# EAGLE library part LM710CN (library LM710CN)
Analog Comparators Source: Datasheet
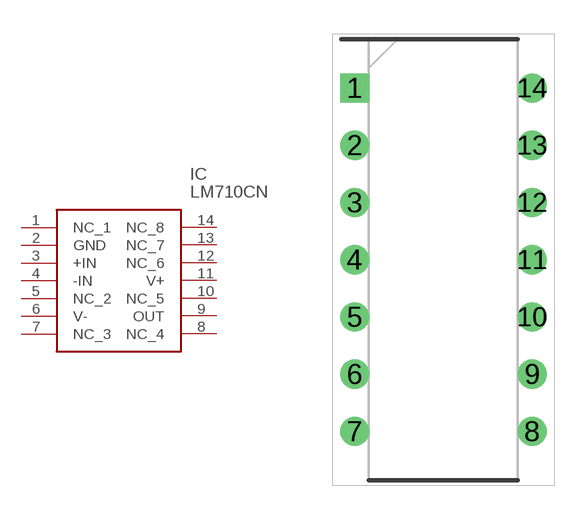
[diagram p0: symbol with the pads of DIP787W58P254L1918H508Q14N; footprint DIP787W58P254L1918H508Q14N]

Designator prefix IC

## LM710CN (Description: Analog Comparators; Height: 5.08mm; Manufacturer_Name: Texas Instruments; Manufacturer_Part_Number: LM710CN; Mouser_Part_Number: N/A; Mouser_Price-Stock: https://www.mouser.com/Search/Refine.aspx?Keyword=N%2FA)  [DIP787W58P254L1918H508Q14N]
1  NC_1
2  GND
3  +IN
4  -IN
5  NC_2
6  V-
7  NC_3
8  NC_4
9  OUT
10  NC_5
11  V+
12  NC_6
13  NC_7
14  NC_8

## Footprint DIP787W58P254L1918H508Q14N (pad centres in mm)
N14A
drill 0.784 pad 1.184 square: 1 -3.937,7.62
drill 0.784 pad 1.184: 2 -3.937,5.08; 3 -3.937,2.54; 4 -3.937,0; 5 -3.937,-2.54; 6 -3.937,-5.08; 7 -3.937,-7.62; 8 3.937,-7.62; 9 3.937,-5.08; 10 3.937,-2.54; 11 3.937,0; 12 3.937,2.54; 13 3.937,5.08; 14 3.937,7.62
